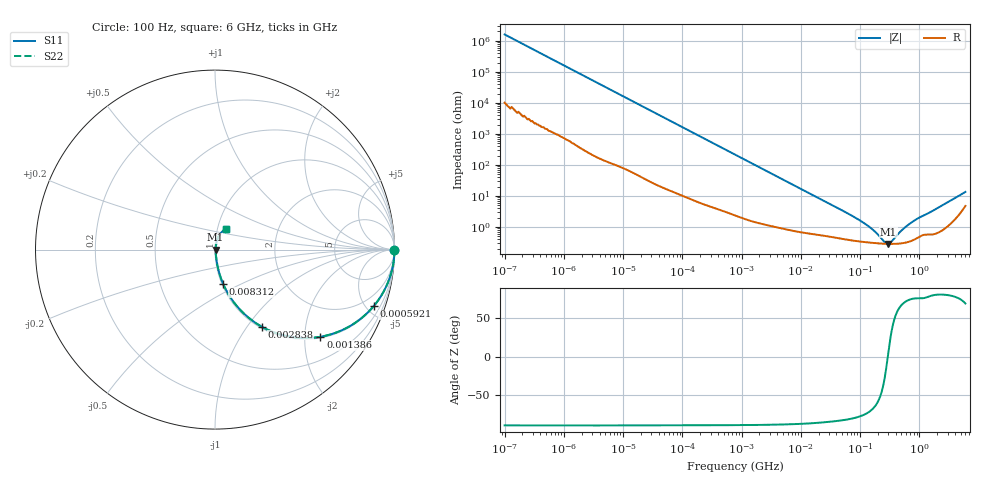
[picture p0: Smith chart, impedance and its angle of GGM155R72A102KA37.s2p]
!Murata Part Number: GGM155R72A102KA37
!These Parameters are Measured in Series Mode Connection
!Data Generated on Jun 19, 2026
!  o--ll--o
!Port1  Port2
!  o------o
!Operation Temp=25[degC], DC Bias Voltage=0[V]
!Freq. Start=100[Hz] Stop=6[GHz] 401[Steps]
# Hz S RI R 50
!Freq.(Hz) S11(Real) S11(Imag) S21(Real) S21(Imag) S12(Real) S12(Imag) S22(Real) S22(Imag)
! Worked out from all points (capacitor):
!   401 points, 100 Hz to 6 GHz, reference 50 ohm
!   read as one part in series: C = 991 pF near 109 Hz
!   lowest |Z| = 286 mohm at 298.8 MHz (marker M1)
!   series resonance near 294 MHz, so ESL is about 300 pH
!   S11 on the Smith chart (normalised r, x): 100 Hz: open; 592.1 kHz: 1.06, -5.57; 1.386 MHz: 1.03, -2.39; 2.838 MHz: 1.02, -1.17; 8.312 MHz: 1.01, -0.40; 6 GHz: 1.10, +0.25
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100  1 -6.24e-05  4e-07 6.24e-05  4e-07 6.24e-05  1 -6.24e-05
171  1 -0.000107  6e-07 0.000107  6e-07 0.000107  1 -0.000107
2008  1 -0.00124  6.6e-06 0.00124  6.6e-06 0.00124  1 -0.00124
40335  0.9993 -0.0247  0.000738 0.0247  0.000738 0.0247  0.9993 -0.0247
184852  0.9867 -0.1111  0.0133 0.1111  0.0133 0.1111  0.9867 -0.1111
361830  0.9522 -0.209  0.0478 0.209  0.0478 0.209  0.9522 -0.209
592111  0.8833 -0.3159  0.1167 0.3159  0.1167 0.3159  0.8833 -0.3159
774597  0.8171 -0.3811  0.1829 0.3811  0.1829 0.3811  0.8171 -0.3811
1386327  0.5872 -0.4857  0.4128 0.4857  0.4128 0.4857  0.5872 -0.4857
1983483  0.4135 -0.4847  0.5865 0.4847  0.5865 0.4847  0.4135 -0.4847
2837864  0.26 -0.4292  0.74 0.4292  0.74 0.4292  0.26 -0.4292
4643984  0.1209 -0.3136  0.8791 0.3136  0.8791 0.3136  0.1209 -0.3136
8311524  0.0456 -0.1916  0.9544 0.1916  0.9544 0.1916  0.0456 -0.1916
1.555665e7  0.0174 -0.1062  0.9826 0.1062  0.9826 0.1062  0.0174 -0.1062
1.066761e8  0.00355 -0.0145  0.9964 0.0145  0.9964 0.0145  0.00355 -0.0145
1.669249e8  0.00311 -0.00734  0.9969 0.00734  0.9969 0.00734  0.00311 -0.00734
2.61201e8  0.00288 -0.00148  0.9971 0.00148  0.9971 0.00148  0.00288 -0.00148
2.987521e8  0.00285 0.000204  0.9972 -0.000204  0.9972 -0.000204  0.00285 0.000204
3.124326e8  0.00284 0.000767  0.9972 -0.000767  0.9972 -0.000767  0.00284 0.000767
5.346885e8  0.00309 0.00807  0.9969 -0.00807  0.9969 -0.00807  0.00309 0.00807
8.000355e8  0.00403 0.015  0.996 -0.015  0.996 -0.015  0.00403 0.015
6e9  0.0593 0.1137  0.9407 -0.1137  0.9407 -0.1137  0.0593 0.1137
